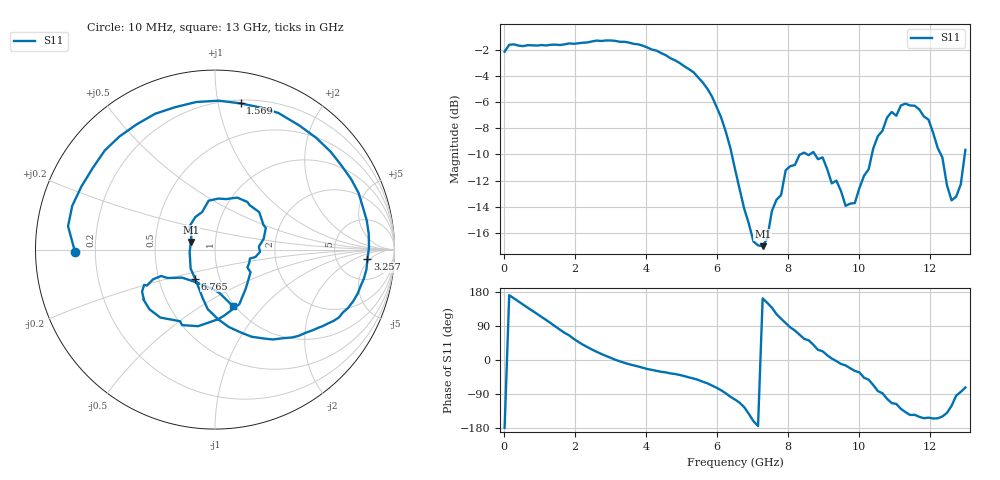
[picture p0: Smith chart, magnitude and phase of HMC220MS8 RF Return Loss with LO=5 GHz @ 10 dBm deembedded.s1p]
!Hittite Microwave Corporation
!12 Elizabeth Drive
!Chelmsford, MA 01824
!Tel: 978-250-3343
!Fax: 978-250-3373
!Device: HMC220MS8, 5-12 GHz, GaAS MMIC SMT Double-Balanced Mixer in 8-lead MSOP package
!Misc: RF Return Loss, LO = 5 GHz @ 10dBm, Room
# MHZ S MA R 50
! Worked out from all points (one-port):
!   101 points, 10 MHz to 13 GHz, reference 50 ohm
!   lowest |S11| = -17.0 dB at 7.284 GHz (marker M1), VSWR 1.33, Z = 38 + j3.26 ohm
!   |S11| at or under -10 dB: 6.414 GHz to 8.35 GHz (1.937 GHz wide, 26.2 % of centre); 8.756 GHz to 10.37 GHz (1.609 GHz wide, 16.8 % of centre); 12.31 GHz to 12.98 GHz (674.8 MHz wide, 5.34 % of centre)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
!   S11 on the Smith chart (normalised r, x): 10 MHz: 0.12, -0.01; 1.569 GHz: 0.23, +1.16; 3.257 GHz: 11, -4; 6.765 GHz: 0.76, -0.26; 13 GHz: 0.98, -0.69
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10  0.78 -179.0
269.8  0.832 163.0
789.4  0.825 130.1
1179.1  0.824 105.7
1568.8  0.827 80.1
1698.7  0.832 71.8
2088.4  0.84 47.9
2478.1  0.854 27.4
3257.5  0.851 -3.5
4036.9  0.809 -23.8
4946.2  0.706 -39.5
5855.5  0.526 -67.3
6505  0.278 -104.4
6764.8  0.196 -124.5
7024.6  0.147 -161.4
7284.4  0.141 162.6
7544.2  0.192 138.2
7933.9  0.275 97.4
8193.7  0.288 77.7
8973.1  0.308 23.2
9752.5  0.205 -21.7
10402  0.333 -66.0
10791.7  0.437 -102.5
11441.2  0.486 -145.0
11960.8  0.429 -152.2
12610.3  0.211 -121.0
12870.1  0.243 -84.1
13000  0.329 -72.6
